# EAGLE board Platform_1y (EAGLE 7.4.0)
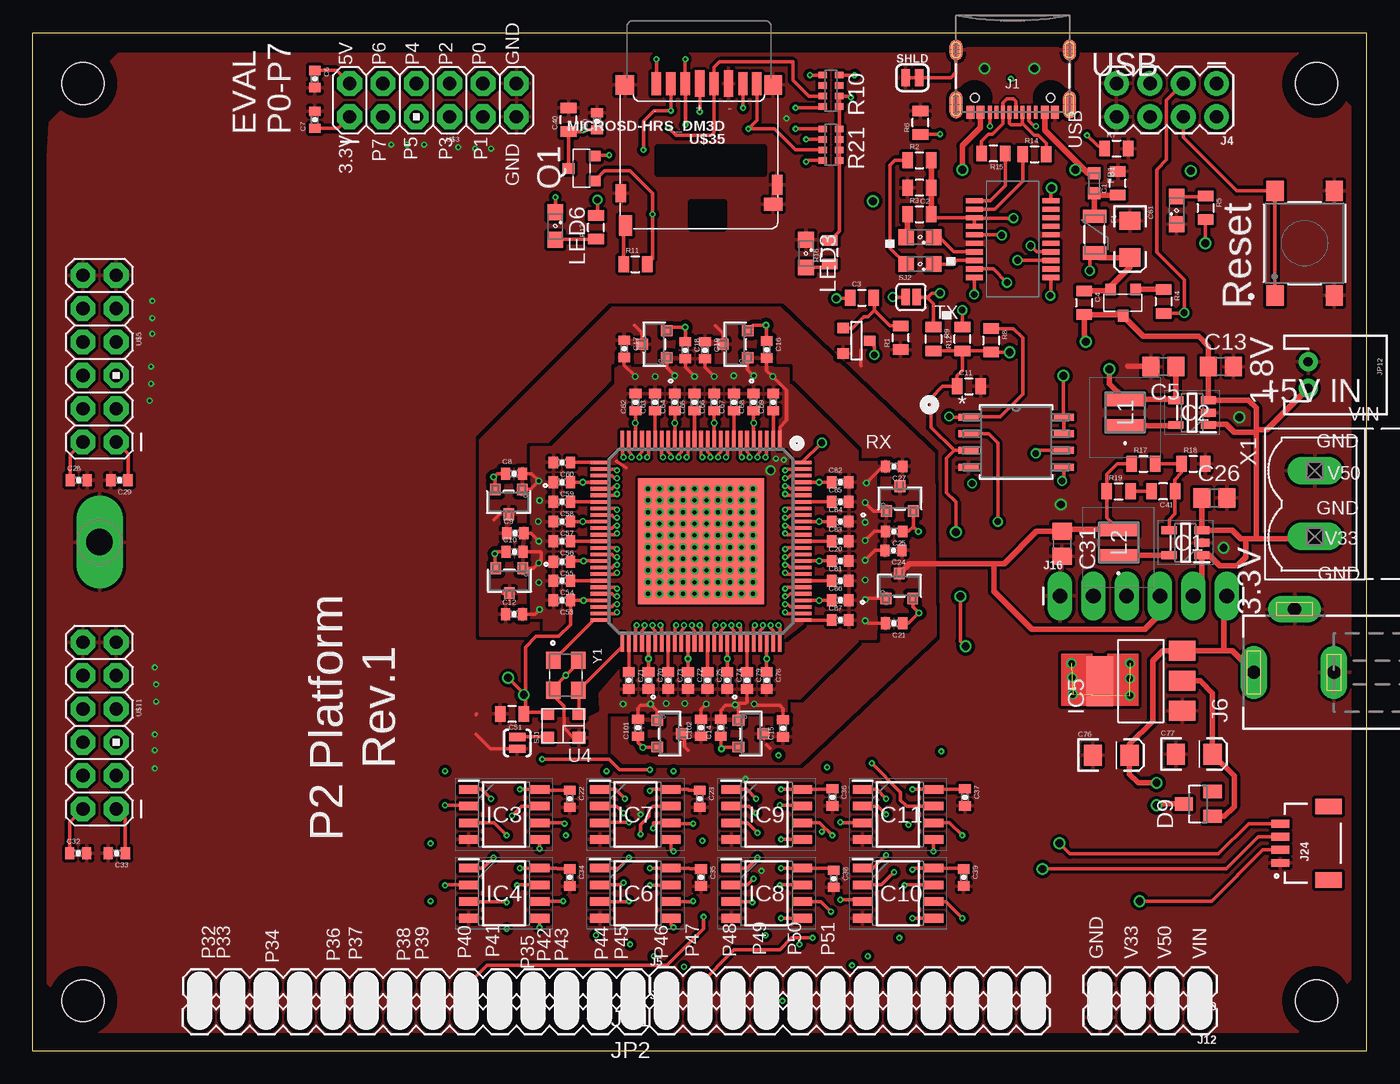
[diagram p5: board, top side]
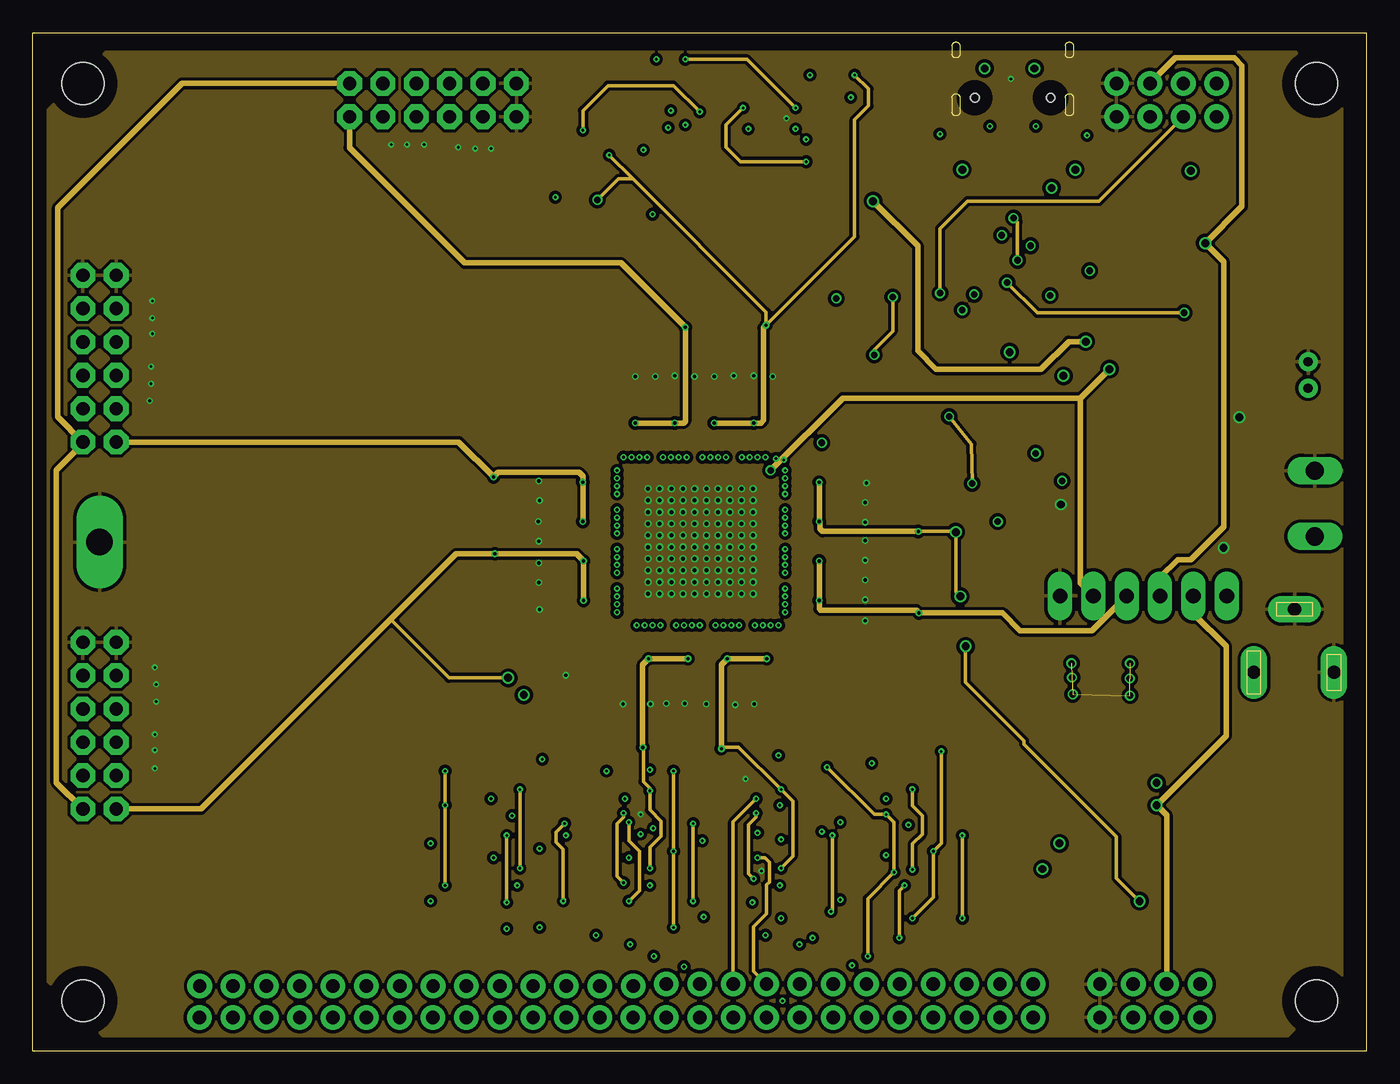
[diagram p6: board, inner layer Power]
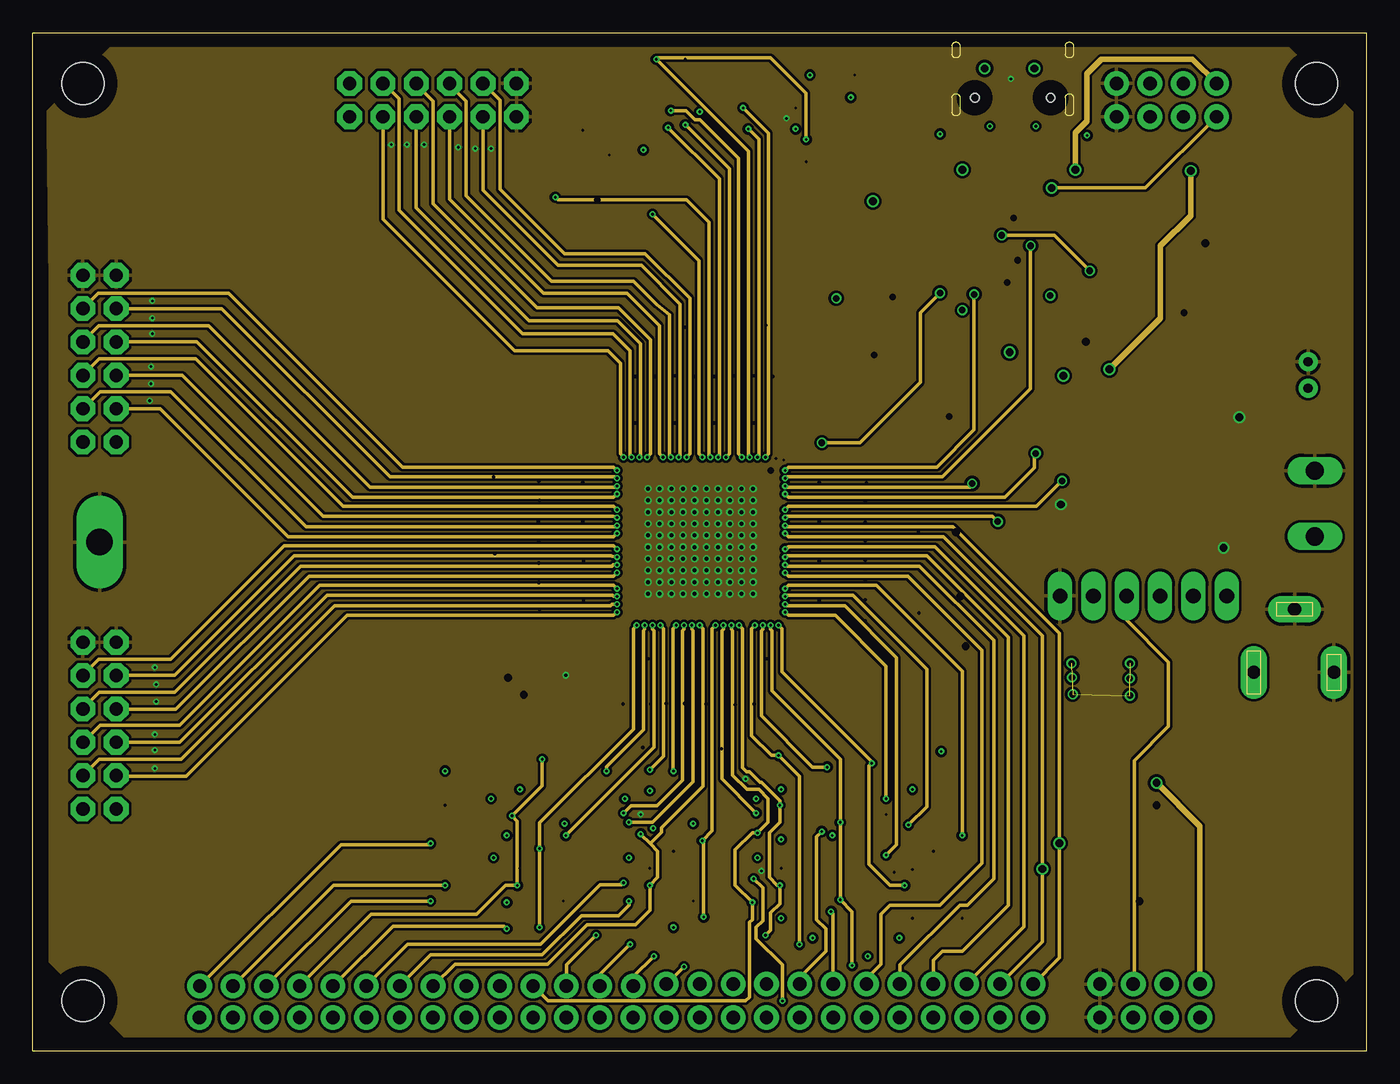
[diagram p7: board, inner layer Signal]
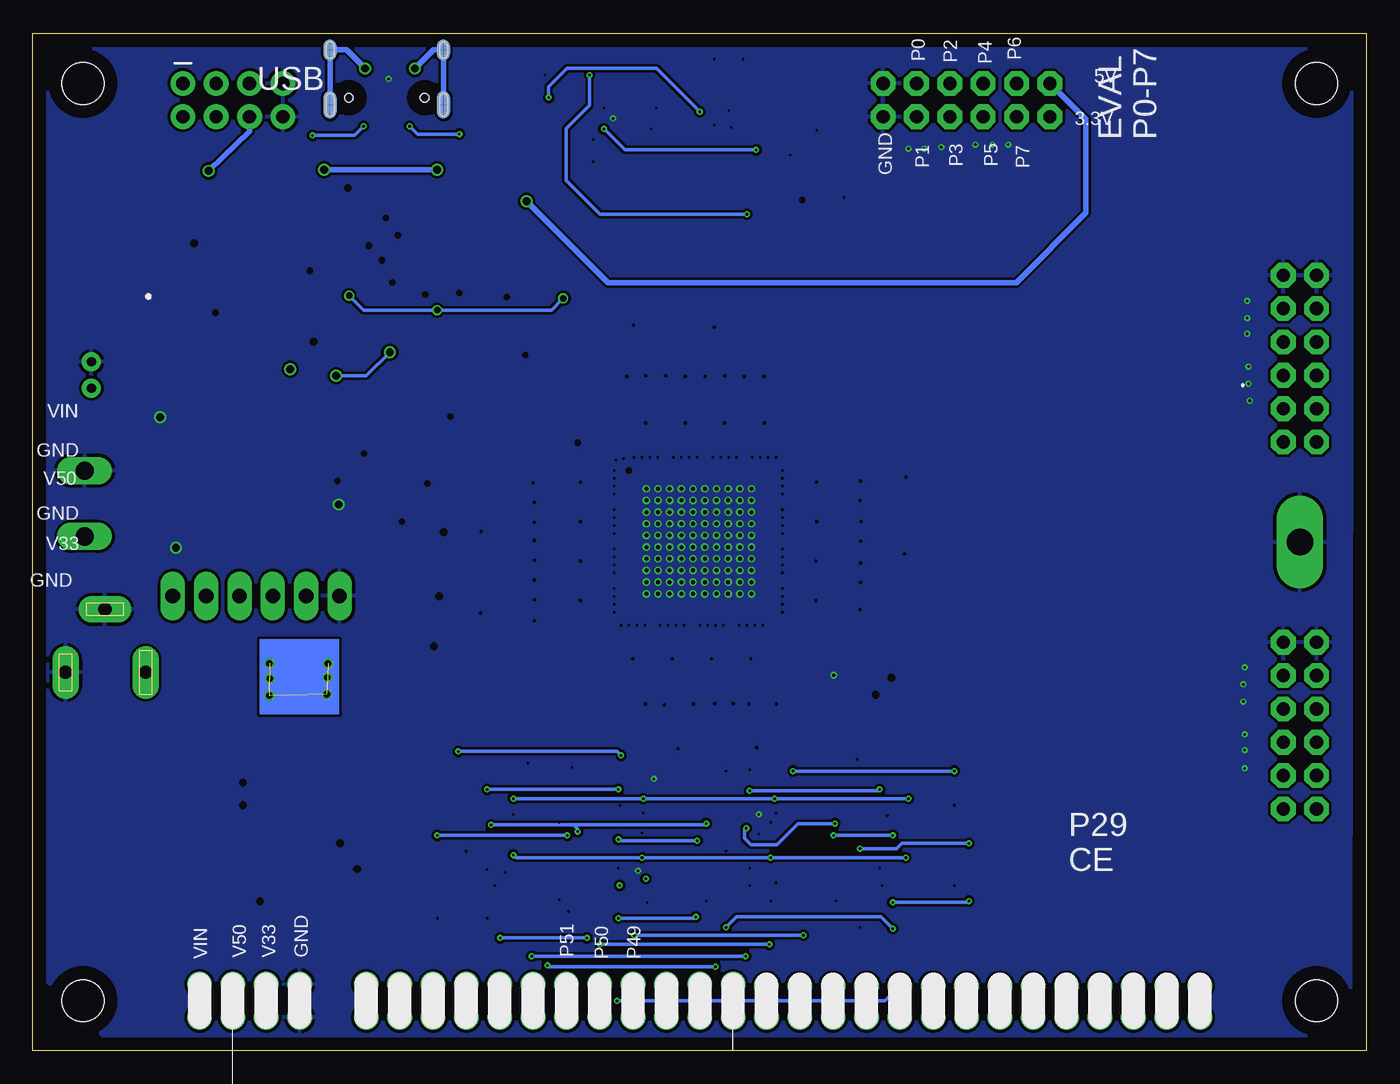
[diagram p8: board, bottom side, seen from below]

Size 101.6 x 77.47 mm. Coordinates in mm from the lower left corner, seen from the top.
Outline: 101.6,0 101.6,77.47 0,77.47 0,0 101.6,0
Copper layers (((1+2)*15)+16): Top 0.035mm / dielectric 1.5mm / Power 0.035mm / dielectric 0.15mm / Signal 0.035mm / dielectric 0.2mm / Bottom 0.035mm
Design rules "default *": minimum track width 5mil, minimum drill 8mil, track to track 6mil, track to pad 6mil, pad to pad 6mil, via to via 6mil, smd to smd 8mil, copper to edge 40mil, drill to drill 8mil, minimum pad ring 4mil, minimum via ring 5mil, stop-mask expansion 4mil, vias tented up to drill 0mil, thermal gap 10mil
Net classes: 0 default: width 0.203 mm, drill 0.406 mm, clearance 0.203 mm; 1 power: width 0.254 mm; 2 gnd: width 0.305 mm, drill 0.406 mm, clearance 0.203 mm
Holes 3.2 mm at 3.81,3.81 3.81,73.66 97.79,73.66 97.79,3.81

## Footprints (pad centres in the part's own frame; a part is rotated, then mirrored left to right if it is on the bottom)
0805 = smd 0.8 x 1.2: 1 -0.9,0; 2 0.9,0
C0805 = smd 1.3 x 1.5: 1 -0.95,0; 2 0.95,0
0402-CAP = smd 0.7 x 0.9: 1 -0.65,0; 2 0.65,0
EIA3216 = smd 1.4 x 1.6: A 1.4,0; C -1.4,0
SOT23 = smd 1 x 1.4: 1 -0.95,-1.1; 2 0.95,-1.1; 3 0,1.1
PTC-1206 = smd 1 x 1.8: 1 -1.4,0; 2 1.4,0
INDC1608X80 = smd 0.92 x 0.98: 1 -0.775,0; 2 0.775,0
SOT95P280X110-5N = smd 1.15 x 0.6: 1 -1.25,0.95; 2 -1.25,0; 3 -1.25,-0.95; 4 1.25,-0.95; 5 1.25,0.95
SOIC127P600X175-8N = smd 1.5 x 0.65: 1 -2.7,1.905; 2 -2.7,0.635; 3 -2.7,-0.635; 4 -2.7,-1.905; 5 2.7,-1.905; 6 2.7,-0.635; 7 2.7,0.635; 8 2.7,1.905
SOT223 = smd 1.499 x 2.007: 1 -2.261,-3.15; 2 0.025,-3.15; 3 2.311,-3.15 | smd 3.81 x 2.007: 4 0,3.15
USB-C-16P-4LAYER-ISOLATED = smd 0.3 x 1: A5 -1.25,-0.34; A6 -0.25,-0.34; A7 0.25,-0.34; A8 1.25,-0.34; B5 1.75,-0.34; B6 0.75,-0.34; B7 -0.75,-0.34; B8 -1.75,-0.34 | smd 0.6 x 1: GND -3.225,-0.34; GND2 3.225,-0.34; VBUS1 -2.45,-0.34; VBUS2 2.45,-0.34 | smd 1 x 2.1: SHLD1 -4.32,-0.915; SHLD2 4.32,-0.915 | smd 1 x 2.1 bottom: SHLD3 -4.32,-0.915; SHLD4 4.32,-0.915 | smd 1 x 1.6: SHLD5 -4.32,-5.095; SHLD8 4.32,-5.095 | smd 1 x 1.6 bottom: SHLD6 -4.32,-5.095; SHLD7 4.32,-5.095 | hole 0.65: -2.89,-1.445; 2.89,-1.445
1X12 = drill 1.016 pad 1.88: 1 0,0; 2 2.54,0; 3 5.08,0; 4 7.62,0; 5 10.16,0; 6 12.7,0; 7 15.24,0; 8 17.78,0; 9 20.32,0; 10 22.86,0; 11 25.4,0; 12 27.94,0
2X4 = drill 1.016 pad 1.88: 1 -3.81,-1.27; 2 -3.81,1.27; 3 -1.27,-1.27; 4 -1.27,1.27; 5 1.27,-1.27; 6 1.27,1.27; 7 3.81,-1.27; 8 3.81,1.27
DCJ0202 = drill 1 pad 2 long: 1 0,3.1; 2 4.8,0; 3 0,-3
1X04 = drill 1.016 pad 1.88: 1 0,0; 2 2.54,0; 3 5.08,0; 4 7.62,0
1X06_LONGPADS = drill 1.118 pad 1.88 long: 1 0,0; 2 2.54,0; 3 5.08,0; 4 7.62,0; 5 10.16,0; 6 12.7,0
JST04_1MM_RA = smd 0.6 x 1.35: 1 -1.5,0; 2 -0.5,0; 3 0.5,0; 4 1.5,0 | smd 1.2 x 2: NC1 2.8,-3.675; NC2 -2.8,-3.675
1X14 = drill 1.016 pad 1.88: 1 0,0; 2 2.54,0; 3 5.08,0; 4 7.62,0; 5 10.16,0; 6 12.7,0; 7 15.24,0; 8 17.78,0; 9 20.32,0; 10 22.86,0; 11 25.4,0; 12 27.94,0; 13 30.48,0; 14 33.02,0
JST-2-PTH = drill 0.7 pad 1.448: 1 -1,0; 2 1,0
VLS3015 = smd 1 x 3: 1 -1,0; 2 1,0
SML0805 = smd 1.2 x 1.2: A 1.05,0; C -1.05,0
MICRO3 = smd 0.8 x 0.9: 1 -0.95,-1; 2 0.95,-1; 3 0,1
0603-ARV = smd 0.5 x 0.65: 1 -1.2,-0.625; 2 -0.4,-0.625; 3 0.4,-0.625; 4 1.2,-0.625; 5 1.2,0.625; 6 0.4,0.625; 7 -0.4,0.625; 8 -1.2,0.625
SMT-JUMPER_2_NC_TRACE_SILK = smd 0.66 x 1.27: 1 -0.521,0; 2 0.521,0
SJ_2S-NO = smd 0.635 x 1.27: 1 -0.45,0; 2 0.45,0
SJ_2S = smd 0.635 x 1.27: 1 -0.412,0; 2 0.412,0
SOT-23 = smd 0.787 x 0.889: 1 0.025,-1.016; 2 -0.94,1.016; 3 0.991,1.016
SSOP20 = smd 0.4 x 1.3: 1 -2.925,-2.925; 2 -2.275,-2.925; 3 -1.625,-2.925; 4 -0.975,-2.925; 5 -0.325,-2.925; 6 0.325,-2.925; 7 0.975,-2.925; 8 1.625,-2.925; 9 2.275,-2.925; 10 2.925,-2.925; 11 2.925,2.925; 12 2.275,2.925; 13 1.625,2.925; 14 0.975,2.925; 15 0.325,2.925; 16 -0.325,2.925; 17 -0.975,2.925; 18 -1.625,2.925; 19 -2.275,2.925; 20 -2.925,2.925
PROPELLER_2 = smd 1.49 x 0.28: 1 -7.67,6; 2 -7.67,5.5; 3 -7.67,5; 4 -7.67,4.5; 5 -7.67,4; 6 -7.67,3.5; 7 -7.67,3; 8 -7.67,2.5; 9 -7.67,2; 10 -7.67,1.5; 11 -7.67,1; 12 -7.67,0.5; 13 -7.67,0; 14 -7.67,-0.5; 15 -7.67,-1; 16 -7.67,-1.5; 17 -7.67,-2; 18 -7.67,-2.5; 19 -7.67,-3; 20 -7.67,-3.5; 21 -7.67,-4; 22 -7.67,-4.5; 23 -7.67,-5; 24 -7.67,-5.5; 25 -7.67,-6; 51 7.67,-6; 52 7.67,-5.5; 53 7.67,-5; 54 7.67,-4.5; 55 7.67,-4; 56 7.67,-3.5; 57 7.67,-3; 58 7.67,-2.5; 59 7.67,-2; 60 7.67,-1.5; 61 7.67,-1; 62 7.67,-0.5; 63 7.67,0; 64 7.67,0.5; 65 7.67,1; 66 7.67,1.5; 67 7.67,2; 68 7.67,2.5; 69 7.67,3; 70 7.67,3.5; 71 7.67,4; 72 7.67,4.5; 73 7.67,5; 74 7.67,5.5; 75 7.67,6 | smd 0.28 x 1.49: 26 -6,-7.67; 27 -5.5,-7.67; 28 -5,-7.67; 29 -4.5,-7.67; 30 -4,-7.67; 31 -3.5,-7.67; 32 -3,-7.67; 33 -2.5,-7.67; 34 -2,-7.67; 35 -1.5,-7.67; 36 -1,-7.67; 37 -0.5,-7.67; 38 0,-7.67; 39 0.5,-7.67; 40 1,-7.67; 41 1.5,-7.67; 42 2,-7.67; 43 2.5,-7.67; 44 3,-7.67; 45 3.5,-7.67; 46 4,-7.67; 47 4.5,-7.67; 48 5,-7.67; 49 5.5,-7.67; 50 6,-7.67; 76 6,7.67; 77 5.5,7.67; 78 5,7.67; 79 4.5,7.67; 80 4,7.67; 81 3.5,7.67; 82 3,7.67; 83 2.5,7.67; 84 2,7.67; 85 1.5,7.67; 86 1,7.67; 87 0.5,7.67; 88 0,7.67; 89 -0.5,7.67; 90 -1,7.67; 91 -1.5,7.67; 92 -2,7.67; 93 -2.5,7.67; 94 -3,7.67; 95 -3.5,7.67; 96 -4,7.67; 97 -4.5,7.67; 98 -5,7.67; 99 -5.5,7.67; 100 -6,7.67 | smd 9.6 x 9.6: EP 0,0
3.2X2.5_4SMD = smd 1 x 0.9: 1 1.2,0.9; 2 -1.2,0.9; 3 -1.2,-0.9; 4 1.2,-0.9
SWITCH_43SMTR92LFS = smd 1.549 x 1.295: 1 -3.975,2.25; 2 3.975,2.25; 3 -3.975,-2.25; 4 3.975,-2.25
SOIC_128JVSIQ_WIN = smd 1.524 x 0.533: 1 -3.645,1.905; 2 -3.645,0.635; 3 -3.645,-0.635; 4 -3.645,-1.905; 5 3.645,-1.905; 6 3.645,-0.635; 7 3.645,0.635; 8 3.645,1.905
SOT-23_DIO = smd 0.813 x 0.889: 1 -1.025,-0.945; 2 1.025,-0.945; 3 0,0.945
6X2HEADER = drill 1.016 pad 1.88 octagon: 1 -1.27,6.35; 2 1.27,6.35; 3 -1.27,3.81; 4 1.27,3.81; 5 -1.27,1.27; 6 1.27,1.27; 7 -1.27,-1.27; 8 1.27,-1.27; 9 -1.27,-3.81; 10 1.27,-3.81; 11 -1.27,-6.35; 12 1.27,-6.35
1X01_TURRET = drill 2.032 pad 3.556 long: 1 0,0
DM3D = smd 0.7 x 1.75: CD/DAT3 8.15,0.45; CLK 4.85,0.45; CMD 7.05,0.45; DAT0 2.65,0.45; DAT1 1.6,0.45; DAT2 9.25,0.45 | smd 0.8 x 1.5: GND1 0.05,8.15 | smd 0.8 x 1.4: GND2 11.95,8.8 | smd 1.4 x 1.5: GND3 11.65,0.55 | smd 1.3 x 1.5: GND4 0.35,0.55 | smd 1 x 1.55: SW_A 11.6,11.25 | smd 1.4 x 1: SW_B 0.35,9.65 | smd 0.7 x 2.032: VDD 5.95,0.45; VSS 3.75,0.45
MSTBV2 = drill 1.397 long: 1 -2.5,0; 2 2.5,0
XTAL_ECS-200-9-33B-CKY-TR = smd 1.3 x 1.1: 1 -1.15,-0.95; 2 1.15,-0.95; 3 1.15,0.95; 4 -1.15,0.95

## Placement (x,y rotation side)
C1  0.1uF  [0805]  82.64,66.06 90 top
C2  0.1uF  [0805]  67.53,65.71 180 top
C3  0.1uF  [0805]  63.15,57.35 0 top
C4  0.1uF  [0805]  80.08,56.96 270 top
C5  4.7u  [C0805]  86.1,52.1 180 top
C6  4.7u  [0402-CAP]  21.48,74 270 top
C7  4.7u  [0402-CAP]  21.48,70.9 90 top
C8  4.7u  [0402-CAP]  36.65,43.95 0 top
C9  4.7u  [0402-CAP]  36.75,39.4 0 top
C10  4.7u  [0402-CAP]  36.7,38 0 top
C11  0.1uF  [0805]  71.3,50.6 0 top
C12  4.7u  [0402-CAP]  36.65,33.25 0 top
C13  4.7u  [C0805]  90.5,52.1 0 top
C14  4.7u  [0402-CAP]  52.4,24.6 90 top
C15  4.7u  [0402-CAP]  57.15,24.55 90 top
C16  4.7u  [0402-CAP]  55.9,53.4 270 top
C17  4.7u  [0402-CAP]  45.05,53.45 270 top
C18  4.7u  [0402-CAP]  49.7,53.35 270 top
C19  4.7u  [0402-CAP]  51.2,53.35 270 top
C20  4.7u  [0402-CAP]  61.5,37.3 0 top
C21  4.7u  [0402-CAP]  65.6,32.55 180 top
C22  4.7u  [0402-CAP]  40.9,19.2 270 top
C23  4.7u  [0402-CAP]  50.8,19.2 270 top
C24  4.7u  [0402-CAP]  65.55,38.1 180 top
C25  4.7u  [0402-CAP]  65.6,39.55 180 top
C26  4.7u  [C0805]  90,42.1 0 top
C27  4.7u  [0402-CAP]  65.6,44.5 180 top
C28  4.7u  [0402-CAP]  3.5,43.45 0 top
C29  4.7u  [0402-CAP]  6.6,43.45 180 top
C30  4.7u  [0402-CAP]  42.98,70.79 90 top
C31  4.7u  [C0805]  78.4,38.6 270 top
C32  4.7u  [0402-CAP]  3.45,15.04 0 top
C33  4.7u  [0402-CAP]  6.4,15.04 180 top
C34  4.7u  [0402-CAP]  40.9,13.2 270 top
C35  4.7u  [0402-CAP]  50.9,13.2 270 top
C36  4.7u  [0402-CAP]  60.9,19.3 270 top
C37  4.7u  [0402-CAP]  71,19.3 270 top
C38  4.7u  [0402-CAP]  61,13.1 270 top
C39  4.7u  [0402-CAP]  70.9,13.2 270 top
C40  0.1uF  [0805]  40.8,70.9 90 top
C41  33p  [0805]  86.1,42.6 180 top
C51  0.1uF  [0805]  36.5,25.65 180 top
C53  4.7u  [0402-CAP]  40.3,34.3 180 top
C54  4.7u  [0402-CAP]  40.3,35.8 180 top
C55  4.7u  [0402-CAP]  40.3,37.25 180 top
C56  4.7u  [0402-CAP]  40.3,38.8 180 top
C57  4.7u  [0402-CAP]  40.3,40.3 180 top
C58  4.7u  [0402-CAP]  40.3,41.8 180 top
C59  4.7u  [0402-CAP]  40.3,43.3 180 top
C60  4.7u  [0402-CAP]  40.3,44.8 180 top
C61  10uF  [EIA3216]  83.58,61.8 270 top
C62  4.7u  [0402-CAP]  45.9,49.4 90 top
C63  4.7u  [0402-CAP]  47.4,49.4 90 top
C64  4.7u  [0402-CAP]  48.9,49.4 90 top
C65  4.7u  [0402-CAP]  50.4,49.4 90 top
C66  4.7u  [0402-CAP]  51.9,49.4 90 top
C67  4.7u  [0402-CAP]  53.4,49.4 90 top
C68  4.7u  [0402-CAP]  54.9,49.4 90 top
C69  4.7u  [0402-CAP]  56.4,49.4 90 top
C70  4.7u  [0402-CAP]  46.9,28.2 270 top
C71  4.7u  [0402-CAP]  45.4,28.2 270 top
C72  4.7u  [0402-CAP]  49.9,28.2 270 top
C73  4.7u  [0402-CAP]  48.4,28.2 270 top
C74  4.7u  [0402-CAP]  52.9,28.2 270 top
C75  4.7u  [0402-CAP]  51.4,28.2 270 top
C76  10uF  [EIA3216]  82.14,22.51 0 top
C77  10uF  [EIA3216]  88.46,22.6 0 top
C78  4.7u  [0402-CAP]  55.9,28.2 270 top
C79  4.7u  [0402-CAP]  54.4,28.2 270 top
C81  4.7u  [0402-CAP]  61.5,35.8 0 top
C82  4.7u  [0402-CAP]  61.5,43.3 0 top
C83  4.7u  [0402-CAP]  61.5,38.8 0 top
C84  4.7u  [0402-CAP]  61.5,40.3 0 top
C85  4.7u  [0402-CAP]  61.5,41.8 0 top
C86  4.7u  [0402-CAP]  61.5,34.3 0 top
C87  4.7u  [0402-CAP]  61.5,32.8 0 top
C101  4.7u  [0402-CAP]  46.1,24.6 90 top
C102  4.7u  [0402-CAP]  50.9,24.6 90 top
D9  BAS40  [SOT23]  88.77,18.8 90 top
F1  500mA  [PTC-1206]  80.88,62.16 270 top
FB1  MPZ1608S221ATA00  [INDC1608X80]  80.83,66.06 270 top
IC1  MCP1603T-330I_OS  [SOT95P280X110-5N]  87.8,38.7 180 top
IC2  MCP1603T-330I_OS  [SOT95P280X110-5N]  88.3,48.6 180 top
IC3  APS6404L-3SQR-SN  [SOIC127P600X175-8N]  35.9,18 0 top
IC4  APS6404L-3SQR-SN  [SOIC127P600X175-8N]  35.9,12 0 top
IC5  REG1117  [SOT223]  84.4,28.16 90 top
IC6  APS6404L-3SQR-SN  [SOIC127P600X175-8N]  45.9,12 0 top
IC7  APS6404L-3SQR-SN  [SOIC127P600X175-8N]  45.9,18 0 top
IC8  APS6404L-3SQR-SN  [SOIC127P600X175-8N]  55.9,12 0 top
IC9  APS6404L-3SQR-SN  [SOIC127P600X175-8N]  55.9,18 0 top
IC10  APS6404L-3SQR-SN  [SOIC127P600X175-8N]  65.9,12 0 top
IC11  APS6404L-3SQR-SN  [SOIC127P600X175-8N]  65.9,18 0 top
J1  USB Female Type C Connector  [USB-C-16P-4LAYER-ISOLATED]  74.64,71.12 180 top
J3  [1X12]  48.26,2.54 0 top
J4  [2X4]  86.36,72.39 180 top
J5  [1X12]  48.26,5.08 0 top
J6  DCJ0202  [DCJ0202]  96.11,28.82 90 top
J10  [1X04]  88.9,5.08 180 top
J12  [1X04]  88.9,2.54 180 top
J16  [1X06_LONGPADS]  78.24,34.63 0 top
J24  QWIIC_RIGHT_ANGLE  [JST04_1MM_RA]  95.03,15.8 90 top
JP1  M14  [1X14]  45.73,4.94 180 top
JP2  M14  [1X14]  45.72,2.54 180 top
JP12  M02JST-PTH-2  [JST-2-PTH]  97.14,51.46 270 top
L1  VLS3015CX-4R7M-1  [VLS3015]  83.2,48.6 90 top
L2  VLS3015CX-4R7M-1  [VLS3015]  82.7,38.7 90 top
LED1  Red  [SML0805]  67.58,59.91 180 top
LED2  Green  [SML0805]  67.58,61.95 180 top
LED3  BLUE  [SML0805]  58.9,60.7 270 top
LED5  Yellow  [SML0805]  87.11,63.99 90 top
LED6  BLUE  [SML0805]  39.8,62.8 270 top
Q1  IRLML5203  [MICRO3]  41.8,67.2 90 top
Q3  IRLML5203  [MICRO3]  83.03,56.97 180 top
R1  10k  [0805]  66.1,54.3 90 top
R2  100  [0805]  67.53,67.81 0 top
R3  100  [0805]  67.53,63.71 0 top
R4  1k  [0805]  86.14,57.06 270 top
R5  100  [0805]  89.33,64.19 270 top
R6  5.1k  [0805]  67.61,70.67 90 top
R7  5.1k  [0805]  82.54,68.7 0 top
R8  10k  [0805]  73,54.1 270 top
R9  10k  [0805]  68.6,54.2 270 top
R10  10k  [0603-ARV]  60.8,73.1 90 top
R11  1k  [0805]  45.9,59.9 0 top
R12  75k  [0805]  70.8,54.2 90 top
R13  1k  [0805]  42.9,62.7 90 top
R14  27  [0805]  76.3,68.27 0 top
R15  27  [0805]  73.17,68.33 180 top
R16  1k  [0805]  60.7,60.8 90 top
R17  200k  [0805]  84.6,44.7 0 top
R18  56.1k  [0805]  88.4,44.7 0 top
R19  5.1k  [0805]  82.7,42.6 0 top
R21  10k  [0603-ARV]  60.8,69 90 top
SHLD  JUMPER-SMT_2_NC_TRACE_SILK  [SMT-JUMPER_2_NC_TRACE_SILK]  67,74.1 0 top
SJ1  SOLDERJUMPERNO  [SJ_2S-NO]  36.9,23.45 270 top
SJ2  SOLDERJUMPERNC  [SJ_2S]  66.9,57.4 0 top
T1  2N3904  [SOT-23]  62.74,54.05 90 top
U1  FT231XS-R  [SSOP20]  74.64,61.81 90 top
U2  Propeller 2 - ES  [PROPELLER_2]  50.9,38.8 270 top
U4  TXEAADSANF-20.000000  [3.2X2.5_4SMD]  40.4,24.75 180 top
U5  PTS645SM43SMTR92LFS  [SWITCH_43SMTR92LFS]  96.87,61.5 90 top
U6  W25Q128JVSIQ  [SOIC_128JVSIQ_WIN]  74.9,46.35 0 top
U$1  AP2120N  [SOT-23_DIO]  36.25,41.8 180 top
U$2  AP2120N  [SOT-23_DIO]  36.3,35.8 180 top
U$3  2X6HEADER  [6X2HEADER]  30.48,72.39 90 top
U$4  AP2120N  [SOT-23_DIO]  48.5,24.15 270 top
U$5  2X6HEADER  [6X2HEADER]  5.08,52.7 180 top
U$6  AP2120N  [SOT-23_DIO]  54.7,24.15 270 top
U$7  AP2120N  [SOT-23_DIO]  53.5,53.8 90 top
U$8  AP2120N  [SOT-23_DIO]  47.35,53.8 90 top
U$9  AP2120N  [SOT-23_DIO]  66,35.4 0 top
U$10  AP2120N  [SOT-23_DIO]  66.05,42.05 0 top
U$11  2X6HEADER  [6X2HEADER]  5.08,24.77 180 top
U$12  [1X01_TURRET]  5.08,38.73 0 top
U$35  MICROSD-HRS_DM3D  [DM3D]  56.74,74.1 180 top
X1  [MSTBV2]  97.65,41.67 270 top
Y1  ECS-200-9-33B-CKY-TR  [XTAL_ECS-200-9-33B-CKY-TR]  40.6,28.6 270 top

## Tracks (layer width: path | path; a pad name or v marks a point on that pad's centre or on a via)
1.8V  (via drill 0.2 layers 1-2, 0.5 layers 1-2, 0.6)
  Top 0.254: 43.23,44.82 U2.26 C60.1 | C71.1 U2.52 | U2.58 C73.1 | U2.64 C75.1 | U2.70 C79.1 | U2.38 C56.1 | U2.32 C58.1 | U2.44 C54.1 | C63.1 U2.20 | C65.1 U2.14 | C67.1 U2.8 | C69.1 U2.2 | C85.1 U2.94 | C83.1 U2.88 | C81.1 U2.82 | C87.1 U2.76 | 44.45,44.9 45.2,44.4
  Top 0.406: L1.2 87,49.6 IC2.4 C5.1 | 83.1,49.7 L1.2 | L1.2 82,50.8 v82,51.9
  Power 0.406: v82,51.9 79.8,49.7 | 79.8,49.7 61.7,49.7 v56.2,44.2 | 79.8,49.7 79.8,35.62 J16.2
  Signal 0.406: v88.2,67 88.2,63.6 85.9,61.3 85.9,55.8 v82,51.9
  Bottom 0.406: v88.2,67 85.09,70.01 J4.6
  other vias: 57.2,45 56.6,45.1
  pour Top (isolate 0.127): 43.85,44.8 44.8,45.75 57.05,45.85 57.8,44.9 58.65,32.5 57.15,31.3 44.85,31.7 43.95,32.7
3V3OUT  (via drill 0.5 layers 1-2)
  Top 0.254: 68.44,63.44 71.2,63.44 | 71.2,63.44 U1.13 U1.14 | U1.3 75.02,60.19 v75,60.2 | v74.7,63.4 71.23,63.4 71.2,63.44
  Top 0.406: R2.2 C2.1 R3.2 68.44,63.44
  Power 0.254: v75,60.2 75,63.1 v74.7,63.4
5V_USB  (via drill 0.5 layers 1-15)
  Top 0.254: 80.5,60.38 v80.5,59.4 | 73.77,62.13 U1.15
  Top 0.406: C4.1 81.97,57.86 Q3.2 82.08,58.18 83.58,59.67 C61.A 81.22,60.41 F1.2 80.5,60.38 | v73.8,62.1 73.77,62.13
  Signal 0.254: v80.5,59.4 77.8,62.1 v73.8,62.1
+5V  (via drill 0.6, 0.6 layers 1-2)
  Top 0.254: U$3.2 23.14,74.65 C6.1 | C28.1 2.85,45.4 U$5.2 | C32.1 2.8,17.41 U$11.2
  Top 0.406: J10.2 J12.2 | C26.1 IC1.3 91.35,39.65 92,39 92.4,39 | IC2.1 89.6,47.7 90.9,47.7 91.5,47.1 93.2,47.1 | D9.3 85.7,18.8 v85.6,18.7 | J16.5 89.05,35.28 IC1.1 89.6,37.75 90.4,36.95 91.75,36.95 92.4,37.6 92.4,39 | X1.2 97.47,39 93.2,39 | 93.2,47.3 93.2,47.1 | 93.2,47.1 93.2,39 | JP12.2 93.97,47.3 93.2,47.3 | v80.2,54 80.08,54.12 C4.2 82.94,56.06 Q3.3 84.6,54.4 88.8,54.4 89.55,53.65 C13.1 IC2.3 92.6,49.55 93.2,48.95 93.2,47.3 | 93.2,39 92.4,39
  Power 0.406: J16.5 88.4,33.3 90.9,30.8 90.9,24 v85.6,18.7 86.36,17.94 J10.2 | v64,64.7 67.4,61.3 67.4,53.3 68.8,51.9 76.8,51.9 78.9,54 v80.2,54 | U$3.2 11.36,73.66 1.9,64.2 1.9,48.27 U$5.2 3.81,46.21 1.8,44.2 1.8,20.43 U$11.2
  Bottom 0.406: v64,64.7 57.8,58.5 26.7,58.5 21.4,63.8 21.4,70.93 U$3.2
BCD  (via drill 0.6 layers 1-15)
  Top 0.254: v77.6,65.7 77.56,65.66 U1.10
  Signal 0.254: J4.2 84.75,65.7 v77.6,65.7
DTR  (via drill 0.5)
  Top 0.254: U1.1 77.56,57.56 v77.5,57.5 | v70.8,56.4 R12.2 | v61.2,57.3 62.2,57.3 C3.1
  Bottom 0.254: v77.5,57.5 76.4,56.4 v70.8,56.4 62.1,56.4 v61.2,57.3
GND  (via drill 0.2, 0.25, 0.25 layers 1-2, 0.3, 0.6)
  Top 0.254: 51.01,39.66 U2.EP 52.03,38.43 | 51.01,39.66 51.34,42.28 49.03,43.43 | Y1.2 39.55,27.45 | 52.03,41.43 53.03,42.43 47.38,42.43 v46.86,41.91 | 49.03,39.43 48.03,40.43 48.03,41.63 v46.86,42.8 | 50.03,40.43 49.03,40.43 49.03,42.43 47.03,42.43 | 50.03,40.43 51.03,40.43 51.03,39.43 | 51.03,39.43 50.03,39.43 | 50.03,40.43 50.03,38.43 48.03,38.43 48.03,39.43 | 47.03,36.43 47.69,35.78 | 47.69,35.78 48.03,35.43 49.03,35.43 49.03,34.43 | 47.03,35.43 47.34,35.43 47.69,35.78 | 49.03,34.43 48.03,34.43 | 54.03,35.43 54.03,34.43 53.03,34.43 | 54.03,35.43 52.03,35.43 52.03,34.43 49.03,34.43 | 54.03,35.43 54.03,37.43 | 51.03,38.43 51.03,37.43 54.03,37.43 | 54.03,37.43 54.03,38 | 54.03,38 54.03,38.43 | 54.03,38.43 55.03,38.43 55.03,34.43 | 54.03,38.43 54.03,39.43 | 54.03,39.43 51.03,39.43 | 54.03,39.43 54.03,41.43 | 54.03,41.43 55.03,41.43 55.03,40.43 | 54.03,41.43 53.03,41.43 | 54.03,41.43 54.03,43.43 | 54.03,43.43 55.03,43.43 55.03,42.43 | 54.03,43.43 53.03,43.43 52.03,42.43 | 63.09,53.4 63.09,52.16 | U$6.1 53.76,26.45 53.75,26.45 54.3,26.45 54.4,26.55 C79.2 | C14.2 52.4,25.95 52.75,26.3 53.45,26.3 v53.5,26.35 | C15.2 57.15,26.05 56.9,26.3 55.05,26.3 v54.95,26.4 | C101.2 46.1,26.1 46.3,26.3 46.95,26.3 v47.05,26.4 47.55,25.89 U$4.1 | C102.2 50.9,26 v51.3,26.4 | Y1.4 41.55,29.55 v40.6,28.6 39.65,27.65 Y1.2 | 33.8,25.65 33.75,25.6 | SJ1.2 34.85,23 33.75,24.1 | U4.2 41.2,23.85 40.45,24.6 40.45,26.25 39.65,27.05 Y1.2 | C12.2 38.25,33.25 v38.6,33.6 | U$2.1 38.15,36.74 v38.55,37.15 38.7,37.3 38.7,37.95 38.65,38 C10.2 | v38.55,38.8 37.95,39.4 C9.2 | U$1.1 37.9,42.74 v38.55,43.4 38,43.95 C8.2 | C17.2 45.05,52.2 v45.9,51.35 | C16.2 55.9,51.8 v56.35,51.35 57.4,50.3 57.4,48 56.9,47.5 U2.1
  Top 0.254: U$7.1 54.45,51.85 v54.9,51.4 | C19.2 51.2,52.05 v51.9,51.35 | C18.2 49.7,52.05 v50.4,51.35 | U$8.1 48.3,52.01 v48.9,51.4 | C21.2 63.6,32.55 v63.4,32.75 | U$9.1 63.51,34.45 v63.4,34.35 | C24.2 64.15,38.1 v63.4,37.35 | C25.2 64.1,39.55 v63.4,38.85 | U$10.1 64.05,41.1 v63.4,41.75 | C27.2 64.75,44.5 v63.5,43.25 | 54.03,38 53.68,38.35 v52.2,38.35 52.2,39.5 51.17,39.5 51.01,39.66
  Top 0.406: C13.2 | IC2.2 | C5.2 83.39,52.11
  other vias: 46.86,34.8 49.65,26.45 48.25,26.45 44.95,26.4 38.55,35.65 38.5,40.3 38.6,41.9 47.4,51.35 53.4,51.4 63.4,40.25 63.4,35.85 47.75,34.8 48.64,34.8 49.53,34.8 50.42,34.8 46.86,35.69 47.75,35.69 48.64,35.69 49.53,35.69 50.42,35.69 46.86,36.58 47.75,36.58 48.64,36.58 49.53,36.58 50.42,36.58 46.86,37.47 47.75,37.47 48.64,37.47 49.53,37.47 50.42,37.47 46.86,38.35 47.75,38.35 48.64,38.35 49.53,38.35 50.42,38.35 46.86,39.24 47.75,39.24 48.64,39.24 49.53,39.24 50.42,39.24 46.86,40.13 47.75,40.13 48.64,40.13 49.53,40.13 50.42,40.13 46.86,41.02 47.75,41.02 48.64,41.02 49.53,41.02 50.42,41.02 47.75,41.91 48.64,41.91 49.53,41.91 50.42,41.91 47.75,42.8 48.64,42.8 49.53,42.8 50.42,42.8 51.31,42.8 52.2,42.8 53.09,42.8 53.98,42.8 54.86,42.8 51.31,41.91 52.2,41.91 53.09,41.91 53.98,41.91 54.86,41.91 51.31,41.02 52.2,41.02 53.09,41.02 53.98,41.02 54.86,41.02 51.31,40.13 52.2,40.13 53.09,40.13 53.98,40.13 54.86,40.13 51.31,39.24 52.2,39.24 53.09,39.24 53.98,39.24 54.86,39.24 51.31,38.35 53.09,38.35 53.98,38.35 54.86,38.35 51.31,37.47 52.2,37.47 53.09,37.47 53.98,37.47 54.86,37.47 51.31,36.58 52.2,36.58 53.09,36.58 53.98,36.58 54.86,36.58 51.31,35.69 52.2,35.69 53.09,35.69 53.98,35.69 54.86,35.69 51.31,34.8 52.2,34.8 53.09,34.8 53.98,34.8 54.86,34.8 9.3,21.5 9.3,22.9 9.3,24.1 9.4,26.6 9.4,27.9 9.3,29.2 8.9,49.5 9,50.8 9,52.1 9.1,54.6 9.1,55.8 9.1,57.1 54.3,20.7 55.5,13.7 46.3,18 27.3,69 28.5,69 29.8,69 32.4,68.8 33.7,68.7 34.9,68.7 74.5,74 78.3,41.6 57.4,71 90.7,38.3 91.9,48.25
  pour Bottom (isolate 0.012): 100.67,75.41 101,5.78 95.45,0.3 3.05,0.5 1.2,4.85 1.1,73.86 5.19,76.71 97.28,76.66
  pour Top: 44.3,27.8 57.3,27.8 57.3,25.9 44.3,25.9 44.3,27.5
  pour Signal: 1.05,70.15 1.05,71.6 6.05,76.6 95.5,76.6 100.7,71.4 100.7,5.95 95.75,1 6.95,1 1.2,6.75 1.2,58.5
  pour Power (isolate 0.254, rank 2): 1.05,71.55 5.55,76.05 96.2,76.05 99.7,72.55 99.7,5.25 95.55,1.1 5.35,1.1 1.1,5.35 1.1,66.35
  pour Top: 40,45.9 38.05,45.85 38.05,33.05 40.1,33.1 40.1,43.85
  pour Top: 44.5,49.75 44.5,51.85 57.45,51.85 57.45,49.65 47.75,49.65
  pour Top: 61.9,44.6 61.9,31.5 64.1,31.5 64.1,44.7 63.2,44.7
  pour Top (isolate 0.254, rank 6): 1.25,70.65 6.55,75.95 96.35,75.95 100.4,71.9 100.4,5.45 96.35,1.4 4.85,1.4 1.1,5.15 1.1,68
N$1
  Top 0.254: 36.85,23.9 SJ1.1 39.15,23.9 U4.1
N$2
  Top 0.254: R2.1 65.66,67.81 65.3,67.45 65.3,61.13 LED1.A
N$3
  cutout Top (isolate 0.305): 38.2,31.1 41.05,31.3 42.55,32.8 43.6,32.8 44.85,31.55 44.8,29.45 42.95,27.25 43,25.95 42.25,25.55 39.2,25.55 38.2,25.95
N$4
  Top 0.406: R3.1 66.64,61.95 LED2.A
N$5  (via drill 0.5 layers 1-2)
  Top 0.254: SJ2.1 v65.5,57.4 | T1.1 63.7,54.01 64.1,53.61 v64.1,53
  Power 0.254: v65.5,57.4 65.5,54.8 64.1,53.4 v64.1,53
N$6  (via drill 0.2)
  Top 0.254: J1.A5 75.89,70.81 76.3,70.4 v76.4,70.4 | v80.3,69.7 v80.31,69.7 81.11,68.91 R7.1
  Bottom 0.254: v76.4,70.4 77.1,69.7 v80.3,69.7
N$7  (via drill 0.2)
  Top 0.254: J1.B5 72.89,70.42 v72.9,70.4 | v69.1,69.8 69.08,69.78 R6.1
  Bottom 0.254: v72.9,70.4 72.3,69.8 v69.1,69.8
N$8
  Top 0.254: C41.2 R19.2
N$9
  Top 0.406: C1.1 80.96,65.16 FB1.2 80.88,65.25 F1.1
N$10
  Top 0.254: U$35.SW_A 45,62.71 R11.1
N$11
  Top 0.254: R14.1 75.39,66.19 73.28,64.08 U1.12
N$12
  Top 0.254: R15.1 74.06,65.86 72.94,64.73 U1.11
N$13
  Top 0.406: IC5.2 88.92,28.18 89.86,27.24 C77.A 91.5,20.96 91.5,18.6 90.75,17.85 D9.1
N$14
  Top 0.254: LED3.A 60.45,59.65 R16.1
N$15
  Top 0.254: J1.B7 75.39,70.61 | 75.39,70.61 76.3,69.7 76.6,69.7 77.19,69.11 R14.2 | J1.A7 74.39,70.61 74.5,70.5 75.27,70.5 75.39,70.61
N$16
  Top 0.254: R15.2 72.27,69.27 72.8,69.8 73.1,69.8 73.89,70.58 J1.B6 73.89,72.19 74.2,72.5 74.7,72.5 74.89,72.31 J1.A6
N$17
  Top 0.406: IC2.5 87,47.6 L1.1
N$18
  Top 0.254: R17.2 R18.1 87.5,44 87,43.5 C41.1 87,40.9 86.55,40.45 IC1.4
N$19
  Top 0.406: IC1.5 82.75,37.75 L2.1
N$24
  Top 0.406: Q3.1 84.07,57.97 84.1,58 86.09,58 R4.1
N$25
  Top 0.254: R1.2 65.3,55.2 64.1,56.4 | 64.1,56.4 64.1,57.3 C3.2 | T1.3 62.44,55.04 63.3,55.9 63.6,55.9 64.1,56.4
N$28
  Top 0.254: LED6.A 39.85,61.8 R13.1
N$45
  Top 0.254: R5.1 89.28,65.05 LED5.A
P0  (via drill 0.2 layers 1-15, 0.2 layers 1-2)
  Top 0.254: U2.3 55.9,45.3 v55.8,45.2 | v54.1,71.8 U$35.DAT0 | R21.8 59,67.8 v58.9,67.7
  Power 0.254: v58.9,67.7 53.9,67.7 52.8,68.8 52.8,70.5 v54.1,71.8
  Signal 0.254: v55.8,45.2 56.05,45.45 56.05,69.85 v54.1,71.8
P1  (via drill 0.2 layers 1-15)
  Top 0.254: U2.4 55.4,45.6 55.2,45.4 v55.2,45.2 | U$35.DAT1 55.14,70.84 v54.5,70.2 56.5,70.2 58.1,68.6 R21.7
  Signal 0.254: v55.2,45.2 55.3,45.3 55.3,69.4 v54.5,70.2
P2  (via drill 0.2 layers 1-15)
  Top 0.254: U2.6 54.4,45.6 54.6,45.4 v54.6,45.2 | v47.5,75.5 U$35.DAT2 | R21.6 v58.9,69.4
  Signal 0.254: v54.6,45.2 54.5,45.3 54.5,68.5 v47.5,75.5 47.6,75.6 56.2,75.6 58.9,72.9 v58.9,69.4
P3  (via drill 0.2, 0.2 layers 1-15)
  Top 0.254: U2.7 53.9,45.3 v54,45.2 | U$35.CD/DAT3 v48.6,71.6 47.3,71.6 46.5,70.8 v46.5,68.6 | R21.5 v58.1,70.2
  Signal 0.254: v54,45.2 53.75,45.45 53.75,67.95 50.8,70.9 50.45,70.9 49.75,71.6 v48.6,71.6
  Bottom 0.254: v58.1,70.2 56.5,68.6 v46.5,68.6
P4  (via drill 0.2 layers 1-15, 0.2 layers 1-2)
  Top 0.254: U2.9 52.9,45.3 v52.8,45.2 | v49.7,70.5 U$35.CMD v49.69,75.49 v49.7,75.5 | R10.8 60.08,71.8 v58.1,71.8
  Power 0.254: v58.1,71.8 54.4,75.5 v49.7,75.5
  Signal 0.254: v52.8,45.2 53.05,45.45 53.05,67.15 v49.7,70.5
P5  (via drill 0.2 layers 1-15)
  Top 0.254: U2.10 52.4,45.6 52.2,45.4 v52.2,45.2 | v48.4,70.3 49,69.7 51.7,69.7 51.89,69.89 U$35.CLK 51.89,74.89 52.3,75.3 57.9,75.3 57.9,73.9 59.1,72.7 R10.7
  Signal 0.254: v52.2,45.2 52.3,45.3 52.3,66.4 v48.4,70.3
P6  (via drill 0.2 layers 1-15)
  Top 0.254: U2.12 51.4,45.6 51.6,45.4 v51.6,45.2 | v39.8,65 LED6.C
  Signal 0.254: v51.6,45.2 51.5,45.3 51.5,63.1 49.8,64.8 40,64.8 v39.8,65
P7  (via drill 0.2, 0.2 layers 1-15)
  Top 0.254: U2.13 50.9,45.3 v51,45.2 | Q1.1 43.55,67 45.5,67 47.2,65.3 v47.2,63.7 47.2,60.3 R11.2 | R10.5 v59.2,74.3
  Signal 0.254: v51,45.2 50.75,45.45 50.75,60.15 v47.2,63.7
  Bottom 0.254: v59.2,74.3 59.2,72 61,70.2 61,66.3 58.4,63.7 v47.2,63.7
P8  (via drill 0.2 layers 1-15)
  Top 0.254: U2.15 49.9,45.3 v49.8,45.2
  Signal 0.254: v49.8,45.2 50.05,45.45 50.05,57.3 46.65,60.7 40.5,60.7 35.6,65.6 35.6,72.4 34.34,73.66 U$3.10
P9  (via drill 0.2 layers 1-15)
  Top 0.254: U2.16 49.4,45.6 49.2,45.4 v49.2,45.2
  Signal 0.254: v49.2,45.2 49.3,45.25 49.3,56.85 46.35,59.8 40,59.8 34.29,65.51 U$3.9
P10  (via drill 0.2 layers 1-15)
  Top 0.254: U2.18 48.4,45.6 48.6,45.4 v48.6,45.2
  Signal 0.254: v48.6,45.2 48.5,45.3 48.5,56.05 47.55,56.8 45.75,58.6 39.5,58.6 33,65.1 33,72.3 31.75,73.55 U$3.8
P11  (via drill 0.2 layers 1-15)
  Top 0.254: U2.19 47.9,45.3 v48,45.2
  Signal 0.254: v48,45.2 47.75,45.45 47.75,55.2 45.25,57.7 38.9,57.7 31.75,64.85 U$3.7
P12  (via drill 0.2 layers 1-15)
  Top 0.254: U2.21 46.9,45.35 v46.8,45.2
  Signal 0.254: v46.8,45.2 47.05,45.45 47.05,54.15 44.6,56.6 38.4,56.6 30.5,64.5 30.5,72.3 29.21,73.59 U$3.6
P13  (via drill 0.2 layers 1-15)
  Top 0.254: U2.22 46.4,45.6 46.2,45.4 v46.2,45.2
  Signal 0.254: v46.2,45.2 46.3,45.35 46.3,53.85 44.55,55.6 37.8,55.6 29.21,64.19 U$3.5
P14  (via drill 0.2 layers 1-15)
  Top 0.254: U2.24 45.4,45.6 45.6,45.4 v45.6,45.2
  Signal 0.254: v45.6,45.2 45.5,45.4 45.5,53.3 44.2,54.6 37.3,54.6 27.9,64 27.9,72.5 26.74,73.66 U$3.4
P15  (via drill 0.2 layers 1-15)
  Top 0.254: U2.25 44.9,45.25 v45,45.2
  Signal 0.254: v45,45.2 44.75,45.45 44.75,52.35 43.8,53.3 36.7,53.3 26.67,63.33 U$3.3
P16  (via drill 0.2 layers 1-15)
  Top 0.254: U2.27 44.4,44.3 v44.5,44.2
  Signal 0.254: v44.5,44.2 44.25,44.45 28.15,44.45 14.9,57.7 5,57.7 U$5.10
P17  (via drill 0.2 layers 1-15)
  Top 0.254: U2.28 44.1,43.8 44.3,43.6 v44.5,43.6
  Signal 0.254: v44.5,43.6 44.3,43.7 27.2,43.7 14.4,56.5 6.37,56.5 U$5.9
P18  (via drill 0.2 layers 1-15)
  Top 0.254: U2.30 44.1,42.8 44.3,43 v44.5,43
  Signal 0.254: v44.5,43 44.35,42.9 25.7,42.9 13.4,55.2 5.04,55.2 U$5.8
P19  (via drill 0.2 layers 1-15)
  Top 0.254: U2.31 44.4,42.3 v44.5,42.4
  Signal 0.254: v44.5,42.4 44.25,42.15 24.35,42.15 12.5,54 6.38,54 U$5.7
P20  (via drill 0.2 layers 1-15)
  Top 0.254: U2.33 44.4,41.3 v44.5,41.2
  Signal 0.254: v44.5,41.2 44.25,41.45 23.65,41.45 12.4,52.7 5.08,52.7 U$5.6
P21  (via drill 0.2 layers 1-15)
  Top 0.254: U2.34 44.1,40.8 44.3,40.6 v44.5,40.6
  Signal 0.254: v44.5,40.6 44.2,40.7 22.1,40.7 11.37,51.44 U$5.5
P22  (via drill 0.2 layers 1-15)
  Top 0.254: U2.36 44.1,39.8 44.3,40 v44.5,40
  Signal 0.254: v44.5,40 44.35,39.9 20.8,39.9 10.5,50.2 5.12,50.2 U$5.4
P23  (via drill 0.2 layers 1-15)
  Top 0.254: U2.37 44.4,39.3 v44.5,39.4
  Signal 0.254: v44.5,39.4 44.25,39.15 19.45,39.15 9.7,48.9 U$5.3
P24  (via drill 0.2 layers 1-15)
  Top 0.254: U2.39 44.4,38.3 v44.5,38.2
  Signal 0.254: v44.5,38.2 44.25,38.45 19.15,38.45 10.5,29.8 5.04,29.8 U$11.10
P25  (via drill 0.2 layers 1-15)
  Top 0.254: U2.40 44.1,37.8 44.3,37.6 v44.5,37.6
  Signal 0.254: v44.5,37.6 44.1,37.65 44.05,37.7 19.9,37.7 10.8,28.6 6.38,28.6 U$11.9
P26  (via drill 0.2 layers 1-15)
  Top 0.254: U2.42 44.1,36.8 44.3,37 v44.5,37
  Signal 0.254: v44.5,37 44.2,37 44.1,36.9 20.4,36.9 10.8,27.3 5.08,27.3 U$11.8
P27  (via drill 0.2 layers 1-15)
  Top 0.254: U2.43 44.4,36.3 v44.5,36.4
  Signal 0.254: v44.5,36.4 44.25,36.15 21.05,36.15 10.9,26 6.38,26 U$11.7
P28  (via drill 0.2 layers 1-15)
  Top 0.254: U2.45 44.4,35.3 v44.5,35.2
  Signal 0.254: v44.5,35.2 44.25,35.45 21.85,35.45 11.2,24.8 5.12,24.8 U$11.6
P29  (via drill 0.2 layers 1-15)
  Top 0.254: U2.46 44.1,34.8 44.3,34.6 v44.5,34.6
  Signal 0.254: v44.5,34.6 44.25,34.6 44.15,34.7 22.4,34.7 11.2,23.5 U$11.5
P30  (via drill 0.2 layers 1-15)
  Top 0.254: U2.48 44.1,33.8 44.3,34 v44.5,34
  Signal 0.254: v44.5,34 44.1,34 44,33.9 23,33.9 11.3,22.2 5.05,22.2 U$11.4
P31  (via drill 0.2 layers 1-15)
  Top 0.254: U2.49 44.4,33.3 v44.5,33.4
  Signal 0.254: v44.5,33.4 44.25,33.15 23.95,33.15 11.7,20.9 6.41,20.9 U$11.3
P32  (via drill 0.2, 0.2 layers 1-15)
  Top 0.254: U2.53 45.9,32.3 v46,32.4 | 38.8,9.9 IC4.5 v38.6,9.4 | v38.6,15.4 IC3.5 | JP1.14 JP2.14
  Signal 0.254: v46,32.4 45.75,32.15 45.75,24.5 38.6,17.35 v38.6,15.4 v38.6,9.4 | JP1.14 23.46,15.7 30.2,15.7 v30.3,15.8
  Bottom 0.254: v30.3,15.8 35.4,15.8 35.8,15.4 v38.6,15.4
P33  (via drill 0.2, 0.2 layers 1-15, 0.2 layers 1-2)
  Top 0.254: U2.54 46.4,32 46.6,32.2 v46.6,32.4 | v31.4,18.7 33.13,18.7 IC3.2 | IC4.2 31.43,12.63 v31.4,12.6 | JP1.13 JP2.13
  Power 0.254: v31.4,21.3 v31.4,18.7 v31.4,12.6
  Signal 0.254: v46.6,32.4 46.6,32.1 46.5,32 46.5,24.45 43.7,21.65 v43.7,21.3 | JP1.13 22.91,12.6 v31.4,12.6
  Bottom 0.254: v43.7,21.3 v31.4,21.3
P34  (via drill 0.2, 0.2 layers 1-15)
  Top 0.254: U2.56 47.4,32 47.2,32.2 v47.2,32.4 | v36.1,16.4 35.13,17.36 IC3.3 | IC4.3 36.03,11.37 v36.1,11.3 | JP1.12 JP2.12
  Power 0.254: v36.1,11.3 v36.1,16.4
  Signal 0.254: v47.2,32.4 47.2,32.1 47.3,32 47.3,23.1 v40.6,16.4 | JP1.12 24.25,11.4 v30.3,11.4
  Bottom 0.254: v40.6,16.4 v36.1,16.4 | v30.3,11.4 30.4,11.3 v36.1,11.3
P35  (via drill 0.2 layers 1-15)
  Top 0.254: U2.57 47.9,32.3 v47.8,32.4 | v47,21.4 44.7,21.4 43.9,22.2 v38.8,22.2 | v36.5,17.9 37.23,18.64 IC3.7 | v36.9,12.6 36.94,12.63 IC4.7 | JP1.11 JP2.11
  Signal 0.254: v47.8,32.4 48.05,32.15 48.05,22.45 v47,21.4 | v38.8,22.2 38.8,20.2 v36.5,17.9 36.9,17.5 v36.9,12.6 36,12.6 33.8,10.4 25.79,10.4 JP1.11
P36  (via drill 0.2, 0.2 layers 1-15, 0.2 layers 1-2)
  Top 0.254: U2.59 48.9,32.3 v49,32.4 | v48.8,15.2 48.6,15.4 IC7.5 | IC6.5 48.6,9.6 v48.8,9.4 | JP1.10 JP2.10
  Power 0.254: v48.8,21.3 v48.8,15.2 v48.8,9.4
  Signal 0.254: v49,32.4 48.75,32.15 48.75,21.35 v48.8,21.3 | JP1.10 27.43,9.5 35.9,9.5 v36.1,9.3 | 48.7,9.5 v48.8,9.4
  Bottom 0.254: v36.1,9.3 37,10.2 48,10.2 v48.8,9.4
P37  (via drill 0.2 layers 1-15)
  Top 0.254: U2.60 49.4,32 49.6,32.2 v49.6,32.4 | 43.23,18.6 IC7.2 44.47,18.64 v45,18.1 | IC6.2 44.84,12.63 v45,12.8 | JP1.9 JP2.9
  Power 0.254: v45,12.8 44.5,13.3 44.5,17.3 45,17.8 v45,18.1
  Signal 0.254: v49.6,32.4 49.6,32.1 49.5,32 49.5,20.6 47.55,18.65 45.55,18.65 v45,18.1 | JP1.9 28.57,8.1 38.66,8.1 IC6.2 44.84,12.63 v45,12.8
P38  (via drill 0.2 layers 1-15)
  Top 0.254: U2.62 50.4,32 50.2,32.2 v50.2,32.4 | 43.16,17.4 IC7.3 43.23,17.4 v45.4,17.4 | IC6.3 45.37,11.37 v45.4,11.4 | JP1.8 JP2.8
  Power 0.254: v45.4,11.4 46.2,12.2 46.2,15.2 45.4,16 v45.4,17.4 45.5,17.4
  Signal 0.254: v50.2,32.4 50.2,32.1 50.3,32 50.3,20.5 47.2,17.4 v45.4,17.4 | JP1.8 30.3,7.3 38.8,7.3 41.8,10.3 44.6,10.3 45.4,11.1 v45.4,11.4
P39  (via drill 0.2 layers 1-15)
  Top 0.254: U2.63 50.9,32.3 v50.8,32.4 | IC6.7 48.47,12.5 48.37,12.6 v47,12.6 | IC7.7 47.23,18.64 46.95,18.35 46.95,17.85 46.3,17.2 v46.3,16.5 | JP1.7 JP2.7
  Signal 0.254: v50.8,32.4 51.05,32.15 51.05,20.15 47.9,17 47.9,16.65 47.05,15.8 47.05,15.75 | v46.3,16.5 47.05,15.75 | 47.05,15.75 47.6,15.2 47.6,13.2 v47,12.6 47,10.7 45.9,9.6 42.2,9.6 39.2,6.6 32.15,6.6 JP1.7
P40  (via drill 0.2, 0.2 layers 1-15)
  Top 0.254: U2.65 51.9,32.3 v52,32.4 | v57,16.1 IC9.5 | IC8.5 v57.01,10.1 v57,10.1 | v51.1,10.2 51.1,9.3 48.3,6.5 34.59,6.5 JP1.6 JP2.6
  Signal 0.254: v52,32.4 51.75,32.15 51.75,16.75 v51,16 51.1,15.9 v51.1,10.2
  Bottom 0.254: v51,16 56.9,16 v57,16.1 | v57,10.1 51.2,10.1 v51.1,10.2
P41  (via drill 0.2, 0.2 layers 1-15)
  Top 0.254: U2.66 52.4,32 52.6,32.2 v52.6,32.4 | v55.1,18.1 54.56,18.64 IC9.2 | IC8.2 54.44,12.63 v54.9,13.1 | JP2.5 JP1.5
  Power 0.254: v54.9,13.1 54.5,13.5 54.5,17.2 55.1,17.8 v55.1,18.1
  Signal 0.254: v52.6,32.4 52.6,32.1 52.5,32 52.5,20.7 v55.1,18.1 | v57.1,3.8 57.1,6.55 55.1,8.55 55.1,9.4 55.6,9.9 55.6,12.4 v54.9,13.1
  Bottom 0.254: JP1.5 36.7,3.8 v57.1,3.8
P42  (via drill 0.2 layers 1-15)
  Top 0.254: U2.68 53.4,32 53.2,32.2 v53.2,32.4 | v55.2,16.6 54.44,17.36 IC9.3 | v54.8,11.3 54.73,11.37 IC8.3 | JP2.4 JP1.4
  Signal 0.254: v53.2,32.4 53.2,32.1 53.3,32 53.3,21 54.4,19.9 55.3,19.9 56,19.2 56,17.4 v55.2,16.6 54.8,16.6 53.5,15.3 53.5,12.6 v54.8,11.3 54.8,10 54.6,9.8 54.6,4.1 54.3,3.8 39.24,3.8 JP1.4
P43  (via drill 0.2, 0.2 layers 1-15)
  Top 0.254: U2.69 53.9,32.3 v53.8,32.4 | v56.9,18.7 58.53,18.7 IC9.7 | IC8.7 56.94,12.63 v56.9,12.6 | JP2.3 JP1.3
  Signal 0.254: v53.8,32.4 54.05,32.15 54.05,21.55 54.35,21.25 54.6,21.25 55.4,20.45 55.5,20.45 56.9,19.05 v56.9,18.7 56.9,17.4 56.1,16.6 56.1,13.2 56.7,12.6 v56.9,12.6 56.9,11.2 56.2,10.5 56.2,9.2 v55.8,8.8 | JP1.3 40.65,6.54 v42.9,8.8
  Bottom 0.254: v42.9,8.8 v55.8,8.8
P44  (via drill 0.2, 0.2 layers 1-15, 0.2 layers 1-2)
  Top 0.254: U2.71 54.9,32.3 v55,32.4 | v68.6,15.2 IC11.5 | IC10.5 v67,10.1 | JP2.2 JP1.2
  Power 0.254: v69.2,22.8 69.2,15.8 v68.6,15.2 68.6,11.7 v67,10.1
  Signal 0.254: v55,32.4 54.75,32.15 54.75,24 56.25,22.5 v56.8,22.5 58.4,20.9 v58.4,8.1 | JP1.2 43.19,5.79 v45.5,8.1
  Bottom 0.254: v56.8,22.5 57.1,22.8 v69.2,22.8 | v45.5,8.1 v58.4,8.1
P45  (via drill 0.2, 0.2 layers 1-15, 0.2 layers 1-2)
  Top 0.254: U2.72 55.4,32 55.6,32.2 v55.6,32.4 | v65,18 64.36,18.64 IC11.2 | IC10.2 64.64,12.63 v65.6,13.6 | JP2.1 JP1.1
  Power 0.254: v60.5,21.6 64.1,18 v65,18 65.6,17.4 v65.6,13.6 63.6,11.6 v63.6,7.2
  Signal 0.254: v55.6,32.4 55.6,32.1 55.5,32 55.5,25.5 59.4,21.6 v60.5,21.6 | JP1.1 45.73,5.62 v47.3,7.2
  Bottom 0.254: v47.3,7.2 v63.6,7.2
P46  (via drill 0.2, 0.2 layers 1-15)
  Top 0.254: U2.74 56.4,32 56.2,32.2 v56.2,32.4 | v61.5,17.4 61.53,17.36 IC11.3 | IC10.3 63.06,11.5 v61.5,11.5 | J3.1 J5.1
  Signal 0.254: v56.2,32.4 56.2,32.1 56.3,32 56.3,27.4 61.5,22.2 v61.5,17.4 v61.5,11.5 62.4,10.6 v62.4,6.5 | J5.1 48.28,5.08 v49.6,6.4
  Bottom 0.254: v49.6,6.4 62.3,6.4 v62.4,6.5
P47  (via drill 0.2, 0.2 layers 1-15)
  Top 0.254: U2.75 56.9,32.3 v56.8,32.4 | v63.9,21.9 66.1,19.7 66.1,19.1 66.56,18.64 IC11.7 | IC10.7 66.44,12.63 v66.4,12.6 | v59.4,8.6 57.8,8.6 56.9,7.7 53.42,7.7 J5.2 J3.2
  Power 0.254: v66,8.6 66,12.2 v66.4,12.6
  Signal 0.254: v56.8,32.4 57.05,32.15 57.05,28.85 63.9,22 v63.9,21.9 63.7,21.7 63.7,14.2 65.3,12.6 v66.4,12.6
  Bottom 0.254: v59.4,8.6 v66,8.6
P48  (via drill 0.2, 0.2 layers 1-15)
  Top 0.254: U2.77 57.4,33.3 v57.3,33.4 | IC3.1 34.2,19.91 v34.9,19.2 | v65,19.2 64.3,19.91 IC11.1 | IC7.1 44.4,19.91 v45.1,19.2 | IC9.1 54.4,19.91 v55.1,19.2 | J3.3 J5.3
  Power 0.254: J5.3 53.34,17.44 v55.1,19.2
  Signal 0.254: v57.3,33.4 57.55,33.15 61.15,33.15 65,29.3 v65,19.2
  Bottom 0.254: v34.9,19.2 v45.1,19.2 v55.1,19.2 v65,19.2
P49  (via drill 0.2, 0.2 layers 1-15)
  Top 0.254: U2.78 57.7,33.8 57.5,34 v57.3,34 | IC4.1 34.3,13.9 v35.1,14.7 | v65,14.9 64,13.9 IC10.1 | IC8.1 54.41,13.9 v55.2,14.7 | IC6.1 44.6,13.9 v45.4,14.7 | J3.4 J5.4
  Power 0.254: J5.4 54.9,6.06 54.9,9.45 55.88,10.43 55.88,12.63 56.1,12.85 56.1,14.35 55.75,14.7 v55.2,14.7
  Signal 0.254: v57.3,34 57.4,33.9 61.85,33.9 65.8,29.95 65.8,15.7 v65,14.9
  Bottom 0.254: v35.1,14.7 v45.4,14.7 v55.2,14.7 64.8,14.7 v65,14.9
P50  (via drill 0.2, 0.2 layers 1-15, 0.2 layers 1-2)
  Top 0.254: U2.80 57.7,34.8 57.5,34.6 v57.3,34.6 | IC3.6 40.44,17.36 v40.5,17.3 | v40.4,11.4 38.63,11.4 IC4.6 | v50.3,17.3 48.66,17.3 IC7.6 47.27,17.36 v47.25,16.95 | IC6.6 50.27,11.37 v50.3,11.4 | J3.5 J5.5
  Power 0.254: 40.5,11.5 v40.4,11.4 40.4,15.35 39.85,15.9 39.85,16.65 v40.5,17.3 | v50.3,11.4 v50.3,17.3
  Signal 0.254: v57.3,34.6 57.4,34.7 62.45,34.7 68.1,29.05 68.1,18.6 v66.7,17.2 | J5.5 58.42,5.62 60.4,7.6 60.4,9.3 59.7,10 59.7,16.3 v60.1,16.7
  Bottom 0.254: v66.7,17.2 60.4,17.2 | 60.4,17.2 50.4,17.2 v50.3,17.3 | v60.1,16.7 60.1,16.9 60.4,17.2 | v40.5,17.3 43.3,17.3 44.9,15.7 46.9,15.7 47.4,16.2 47.4,16.9 v47.25,16.95
P51  (via drill 0.2, 0.2 layers 1-15, 0.2 layers 1-2)
  Top 0.254: U2.81 57.4,35.3 v57.3,35.2 | IC9.6 59.94,17.36 v60.9,16.4 | v70.8,16.4 69.83,17.36 IC11.6 | v70.8,10.1 69.53,11.37 IC10.6 | v60.8,10.6 60.03,11.37 IC8.6 | J3.6 J5.6
  Power 0.254: v70.8,16.4 v70.8,10.1 | v60.9,16.4 60.9,10.7 v60.8,10.6
  Signal 0.254: v57.3,35.2 57.55,35.45 64.25,35.45 70.8,28.9 v70.8,16.4 | J5.6 60.96,10.44 v60.8,10.6
  Bottom 0.254: v60.9,16.4 v70.8,16.4
P52  (via drill 0.2 layers 1-15)
  Top 0.254: U2.83 57.4,36.3 v57.3,36.4 | J3.7 J5.7
  Signal 0.254: v57.3,36.4 57.55,36.15 66.65,36.15 72.3,30.5 72.3,14.3 69.1,11.1 65.3,11.1 64.6,10.4 64.6,6.6 63.5,5.5 J5.7
P53  (via drill 0.2 layers 1-15)
  Top 0.254: U2.84 57.7,36.8 57.5,37 v57.3,37 | J3.8 J5.8
  Signal 0.254: v57.3,37 57.4,36.9 67.55,36.9 73.2,31.25 73.2,13.1 71.2,11.1 70.6,11.1 66.04,6.54 J5.8
P54  (via drill 0.2 layers 1-15)
  Top 0.254: U2.86 57.7,37.8 57.5,37.6 v57.3,37.6 | J3.9 J5.9
  Signal 0.254: v57.3,37.6 57.4,37.7 68.1,37.7 74.3,31.5 74.3,11.1 70.8,7.6 69.3,7.6 68.58,6.88 J5.9
P55  (via drill 0.2 layers 1-15)
  Top 0.254: U2.87 57.5,38.3 v57.3,38.2 | J3.10 J5.10
  Signal 0.254: v57.3,38.2 57.6,38.4 68.7,38.4 75.5,31.6 75.5,9.46 J5.10
P56  (via drill 0.2 layers 1-15, 0.6 layers 1-15)
  Top 0.254: U2.89 57.4,39.3 v57.3,39.4 | J3.11 J5.11 | J24.3 93.36,16.3 90.9,13.85 v76.9,13.85
  Signal 0.254: v57.3,39.4 57.55,39.15 69.35,39.15 76.9,31.6 v76.9,13.85 76.9,13.75 76.9,8.32 J5.11
P57  (via drill 0.2 layers 1-15, 0.6 layers 1-15)
  Top 0.254: U2.90 57.7,39.8 57.5,40 v57.3,40 | J3.12 J5.12 | J24.4 92.61,17.3 90.3,15 79,15 v78.2,15.8
  Signal 0.254: v57.3,40 57.4,39.9 70.1,39.9 78.2,31.8 78.2,15.95 v78.2,15.8 78.2,7.08 J5.12
P58_FDO  (via drill 0.2 layers 1-15, 0.5 layers 1-15)
  Top 0.254: U2.92 57.7,40.8 57.5,40.6 v57.3,40.6 | v73.5,40.3 73.5,46.3 72.81,46.98 U6.2
  Signal 0.254: v57.3,40.6 57.4,40.7 73.1,40.7 v73.5,40.3
P59_FDI  (via drill 0.2 layers 1-15, 0.5 layers 1-15)
  Top 0.254: U2.93 57.4,41.3 v57.3,41.2 | v78.4,43.4 78.55,43.55 U6.5
  Signal 0.254: v57.3,41.2 57.55,41.45 76.45,41.45 v78.4,43.4
P60_FCLK  (via drill 0.2 layers 1-15, 0.5 layers 1-15)
  Top 0.254: U2.95 57.4,42.3 v57.3,42.4 | U6.6 76.61,45.72 v76.4,45.5
  Signal 0.254: v57.3,42.4 57.55,42.15 74.05,42.15 76.3,44.4 76.3,45.4 v76.4,45.5
P61_FCSN  (via drill 0.2 layers 1-15, 0.5 layers 1-15, 0.5 layers 1-2)
  Top 0.254: U2.96 57.7,42.8 57.5,43 v57.3,43 | R8.1 74.7,55 75.4,54.3 75.4,50 73.7,48.3 71.3,48.3 U6.1 69.84,48.26 v69.8,48.3
  Power 0.254: v71.55,43.2 71.5,46.2 v69.8,48.3
  Signal 0.254: v57.3,43 57.4,42.9 71.4,42.9 v71.55,43.2
P62_TXD  (via drill 0.2 layers 1-15, 0.5 layers 1-15)
  Top 0.254: U2.98 57.7,43.8 57.5,43.6 v57.3,43.6 | U1.4 76.47,60.84 v76,61.3
  Signal 0.254: v57.3,43.6 57.4,43.7 69.3,43.7 76,50.4 v76,61.3
P63_RXD  (via drill 0.2 layers 1-15, 0.5 layers 1-15)
  Top 0.254: U2.99 57.4,44.3 v57.3,44.2 | v71.7,57.6 v71.71,57.61 U1.20
  Signal 0.254: v57.3,44.2 57.55,44.45 68.85,44.45 71.7,47.3 v71.7,57.6
PWREN  (via drill 0.5 layers 1-2)
  Top 0.254: U1.19 73.17,59.53 v74.2,58.5 | R4.2 87.66,56.16 v87.7,56.2 87.7,58.7 85.6,60.8 85.6,67.1 86.35,67.85 86.35,72.38 J4.3
  Power 0.254: v74.2,58.5 76.5,56.2 v87.7,56.2
RST  (via drill 0.5 layers 1-15)
  Top 0.254: SJ2.2 68.1,57.4 68.15,57.35 | 68.15,57.35 68.6,56.9 R9.1 | U2.100 58.6,44.8 v60.1,46.3 | v69.1,57.7 68.5,57.7 68.15,57.35 | J4.4 87.63,69.57 91.72,65.47 U5.2 U5.1
  Power 0.254: J4.4 81.21,64.7 71.2,64.7 69.1,62.6 v69.1,57.7
  Signal 0.254: v60.1,46.3 63,46.3 67.6,50.9 67.6,56.2 v69.1,57.7
RXLED
  Top 0.254: 69.05,61.95 70.17,60.84 U1.17
  Top 0.406: LED2.C 69.05,61.95
SHLD  (via drill 0.6)
  Top 0.254: SHLD.2 69.92,74.1 70.31,74.5 J1.SHLD8
  Bottom 0.406: v72.5,74.8 71.08,76.22 J1.SHLD8 J1.SHLD2 | v76.3,74.8 77.72,76.22 J1.SHLD5 J1.SHLD1
  pour Top: 70.3,76.3 79,76.3 79,72 70.3,72
THERMAL  (via drill 0.5)  (5 unrouted)
  other vias: 83.56,28.35 79.16,28.43 79.12,29.51 83.58,27.05 83.58,29.5 79.2,27.15
TXLED
  Top 0.254: LED1.C 70.11,59.91 70.39,60.19 U1.18
VBUS  (via drill 0.6)
  Top 0.254: 80.36,66.83 FB1.1 | v79.4,67.1 79.5,67.1 79.8,67.4
  Top 0.406: J1.VBUS1 77.08,70.11 79.8,67.4 80.36,66.83 | J1.VBUS2 72.19,70.28 70.8,68.9 v70.8,67.1
  Signal 0.406: J4.1 88.33,75.5 81.4,75.5 80.3,74.4 80.3,70.8 79.4,69.9 v79.4,67.1
  Bottom 0.406: v70.8,67.1 v79.4,67.1
VIO  (via drill 0.6 layers 1-2)
  Top 0.254: 55.9,23.9 U$6.3 | 55.9,23.3 56.15,23.05 | U$4.3 49.65,23.95 49.65,23.16 49.9,22.9 | U$2.3 35.8,34.85 | 35.15,40.45 35.55,40.85 | 52,55.2 52.55,54.65 U$7.3 52.45,53.9 | 45.85,55.25 46.41,54.7 U$8.3 | L2.2 81.8,40.6 R19.1 81.8,43.9 82.6,44.7 R17.1 | R5.2 89.3,63.26 v89.3,61.5
  Top 0.406: L2.2 78.55,39.7 C31.1 76.45,39.55 74,37.1 73.3,37.1 | 73.3,37.1 66.75,37.1 U$9.3 | 73.3,37.1 73.2,37 73.2,35 76.1,32.1 84.7,32.1 85.86,33.26 J16.4
  Power 0.406: J16.4 85.86,36.06 87.2,37.4 88.2,37.4 90.7,39.9 90.7,60.1 v89.3,61.5 92.1,64.3 92.1,75 91.5,75.6 87.03,75.6 J4.5
  pour Top (isolate 0.305, rank 3): 44.15,21.9 58.4,21.9 68.7,31.6 68.6,45.45 56.9,56.55 44.15,56.55 34.1,46.5 34.1,31.65 38.5,31.65 38.5,45.65 44,51.15 58.05,51.15 63.25,45.95 63.25,30.9 58.75,26.4 44.15,26.4
VIO_0-7  (via drill 0.2 layers 1-2, 0.25 layers 1-2, 0.5 layers 1-2)
  Top 0.254: U2.11 v51.9,47.8 C66.1 | C68.1 v54.9,47.8 | 54.9,47.75 U2.5 | C16.1 55.9,55.2 v55.85,55.25 54.87,55.25 U$7.2 | 42.98,68.33 Q1.2 42.85,68.2 v43.9,68.2 | 61.3,74.3 R10.4 v62.6,74.3 | R13.2 43,63.7 v43,64.8
  Top 0.406: v54.9,47.8 54.9,47.75
  Power 0.254: v43.9,68.2 45.7,66.4 | 45.7,66.4 55.85,56.25 v55.85,55.25 62.6,62 62.6,70.9 63.65,71.95 63.65,73.25 v62.6,74.3 | v43,64.8 44.6,66.4 45.7,66.4
  Power 0.406: v55.85,55.25 55.65,55.05 55.65,48 55.45,47.8 v54.9,47.8 v51.9,47.8
VIO_8-15  (via drill 0.25 layers 1-2)
  Top 0.254: U2.23 v45.9,47.8 C62.1 | C64.1 v48.9,47.8 | 48.9,47.75 U2.17 | C18.1 v49.7,55.1 48.57,55.1 U$8.2 | C7.1 23.26,70.25 U$3.1
  Top 0.406: v48.9,47.8 48.9,47.75
  Power 0.406: v45.9,47.8 v48.9,47.8 49.55,47.8 49.7,47.95 v49.7,55.1 44.8,60 32.9,60 24.13,68.77 U$3.1
VIO_16-23  (via drill 0.25 layers 1-2)
  Top 0.254: U2.35 v41.9,40.3 C57.1 | U2.29 v41.9,43.3 C59.1 | C8.1 35.35,43.95 v35.1,43.7 35.23,43.58 U$1.2 | C29.1 7.25,45.45 U$5.1
  Power 0.406: v41.9,40.3 v41.9,43.3 41.9,43.75 41.6,44.05 35.45,44.05 v35.1,43.7 32.45,46.35 U$5.1
VIO_24-31  (via drill 0.25 layers 1-2, 0.6 layers 1-2)
  Top 0.254: U2.47 v41.95,34.3 C53.1 40.95,32.45 40.05,31.55 38.35,31.55 37.55,30.75 37.55,25.8 | U2.41 v41.95,37.3 41,37.3 C55.1 | 37.55,25.8 C51.1 | 37.55,25.8 39.05,25.8 U4.4 | C10.1 35.35,38 v35.2,37.85 35.2,36.82 U$2.2 | C33.1 7.05,17.71 U$11.1 | v37.4,27.1 37.4,27.2 v36.2,28.4
  Power 0.254: v36.2,28.4 31.7,28.4 27.25,32.85
  Power 0.406: v41.95,34.3 v41.95,37.3 41.45,37.8 41.45,37.85 v35.2,37.85 32.25,37.85 27.25,32.85 12.81,18.41 U$11.1 | 37.3,27.2 v37.4,27.1
VIO_32-39  (via drill 0.2, 0.2 layers 1-2, 0.25 layers 1-2)
  Top 0.254: U2.55 v46.9,29.85 C70.1 | U2.61 v49.9,29.85 C72.1 | U$4.2 46.48,23.12 v46.45,23.1 46.1,23.45 | C101.1 46.1,23.45 | C23.1 49.95,19.85 49.9,19.91 IC7.8 47.1,19.91 v47,19.8 | C35.1 50.05,13.85 49.99,13.9 IC6.8 v47,13.9 | C34.1 39.95,13.85 39.9,13.9 IC4.8 v37.1,13.9 | 46.1,23.45 46.15,23.45 v46.5,23.1 | v37.1,19.9 IC3.8 38.66,19.85 C22.1
  Power 0.254: 46.95,29.85 v46.9,29.85 | v46.5,23.1 46.5,20.5 47,20 v47,19.8 47,18.35 47.85,17.5 47.85,16.35 47,15.5 v47,13.9 | v37.1,13.9 v37.1,19.9
  Power 0.406: v46.45,23.1 46.45,29.4 v46.9,29.85 | v49.9,29.85 46.95,29.85
  Bottom 0.254: v47,19.8 37.2,19.8 v37.1,19.9
VIO_40-47  (via drill 0.2, 0.2 layers 1-2, 0.25 layers 1-2)
  Top 0.254: U2.73 v55.9,29.85 C78.1 | C74.1 v52.9,29.85 U2.67 | C14.1 52.4,23.05 v52.45,23 52.58,23.12 U$6.2 | v57,19.9 v57.01,19.91 IC9.8 60.85,19.91 C36.1 | C37.1 70.95,19.91 IC11.8 v67,19.91 v67,19.9 | C38.1 60.84,13.9 IC8.8 v57.01,13.9 v57,13.9 | C39.1 70.84,13.9 IC10.8 67.11,13.9 v67,13.8
  Power 0.254: v52.45,23 52.58,23.12 U$6.2 56.98,19.9 v57,19.9 57.9,19 57.9,14.8 v57,13.9 | 66.9,20 v67,19.9 67,18.65 67.75,17.9 67.75,16.5 67,15.75 v67,13.8
  Power 0.406: v52.45,23 52.45,29.4 v52.9,29.85 v55.9,29.85
  Bottom 0.254: v67,19.9 v57,19.9
VIO_48-55  (via drill 0.25 layers 1-2)
  Top 0.254: U2.85 v59.9,37.3 C20.1 | U2.79 v59.9,34.3 C86.1 | U$9.2 67.03,33.83 v67.5,33.35 66.7,32.55 C21.1
  Top 0.406: J12.3 J10.3
  Power 0.406: v59.9,37.3 v59.9,34.3 59.9,33.65 60,33.55 67.3,33.55 v67.5,33.35 73.85,33.35 75.2,32 80.69,32 J16.3
  Signal 0.254: J10.3 83.9,5.16 83.9,22.1 86.5,24.7 86.5,29.6 83.32,32.78 J16.3
VIO_56-63  (via drill 0.25 layers 1-2, 0.6, 0.6 layers 1-2)
  Top 0.254: C82.1 v59.9,43.3 U2.97 | U2.91 v59.9,40.3 C84.1 | U$10.2 67.08,39.92 | 67.08,39.92 v67.45,39.55 | R12.1 72.9,53.3 R8.2 v74.4,53.2 | 78.44,51.34 v78.5,51.4 78.5,48.3 U6.8 U6.7 | R12.1 70.8,51.8 70.4,51.4 C11.1 69.3,50.6 68.4,49.7 68.4,47.5 70.19,45.72 | 70.19,45.72 U6.3 | 70.19,45.72 69.6,45.13 69.6,42.5 70.3,41.8 v70.3,39.5 | C25.1 66.7,39.55 67.08,39.92 | R9.2 R12.1 | v70.65,34.6 70.65,31.2 v71.05,30.8 | v84.3,11.4 89.8,11.4 93.7,15.3 J24.2
  Power 0.254: v67.45,39.55 70.25,39.55 v70.3,39.5 70.3,34.95 v70.65,34.6 | v71.05,30.8 71.05,28.05 75.5,23.6 75.5,23.35 82.55,16.3 82.55,13.15 v84.3,11.4
  Power 0.406: v67.45,39.55 60.15,39.55 59.95,39.75 59.95,40.25 v59.9,40.3 v59.9,43.3
  Bottom 0.254: v78.5,51.4 76.2,51.4 v74.4,53.2
VSD  (via drill 0.2, 0.2 layers 1-2)
  Top 0.254: R16.2 61.42,62.42 R21.1 R21.2 R21.3 R21.4 R10.1 R10.2 62.2,72.7 v62.3,72.6 | U$35.VDD v50.8,71.5 | C30.1 41.94,70.14 v41.9,70.1 41.8,70 C40.1 Q1.3
  Power 0.254: v50.8,71.5 48.8,73.5 43.8,73.5 41.9,71.6 v41.9,70.1
  Bottom 0.254: v50.8,71.5 54.1,74.8 60.9,74.8 62.3,73.4 v62.3,72.6
WALL_POWER  (via drill 0.6 layers 1-15)
  Top 0.406: J10.1 J12.1 | J6.1 91.36,30.47 90.7,30.47 | 90.7,30.47 IC5.3 86.07,30.47 85.3,29.7 85.3,25.1 83.54,23.34 C76.A 83.54,21.06 84.2,20.4 v85.6,20.4 | J16.6 90.7,34.4 90.7,30.47
  Signal 0.406: J10.1 88.9,17.1 v85.6,20.4
XI
  Top 0.254: U2.51 44.9,30.8 Y1.3 41.6,27.4 U4.3
XO
  Top 0.254: U2.50 42.7,32.8 Y1.1
(copper drawn outside any net)
  shapes: Bottom area x1, Top area x2

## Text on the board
tPlace: Rev. 1 / Copying Eval.Rev.B / Add solder bridge for USB reset / Add FT231X battery charge signal on new header | VIN | 5V | P6 | P4 | P2 | P0 | GND | USB | LIPO | EVAL / P0-P7 | 3.3V | P5 | P3 | P1 | P7 | GND | USB | +6-9 VDC | Reset | TX | +5V IN | 1.8V | VIN | GND | RX | V50 | GND | V33 | GND | 3.3V | Rev.1 | P2 Platform | P32 | P33 | P34 | P36 | P37 | P38 | P39 | P40 | P41 | P42 | P43 | P44 | P45 | P46 | P47 | P48 | P49 | P50 | P51 | GND | V33 | V50 | VIN | P35
bPlace: P6 | P4 | P2 | P0 | VIN | 5V | USB | 3.3V | +5V IN | EVAL / P0-P7 | P7 | P5 | P3 | P1 | GND | LIPO | VIN | GND | V50 | GND | V33 | GND | P29 / CE | P49 | P50 | P51 | GND | V33 | V50 | VIN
